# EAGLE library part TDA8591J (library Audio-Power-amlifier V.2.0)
The TDA8591J is a quad BTL audio power amplifier comprising four independent amplifiers in Bridge Tied Load (BTL) configuration. Each amplifier has a gain of 26 dB and supplies an output power of 75 W (EIAJ) into a 2 W load. The TDA8591J has low quiescent current and is primarily developed for car audio applications.
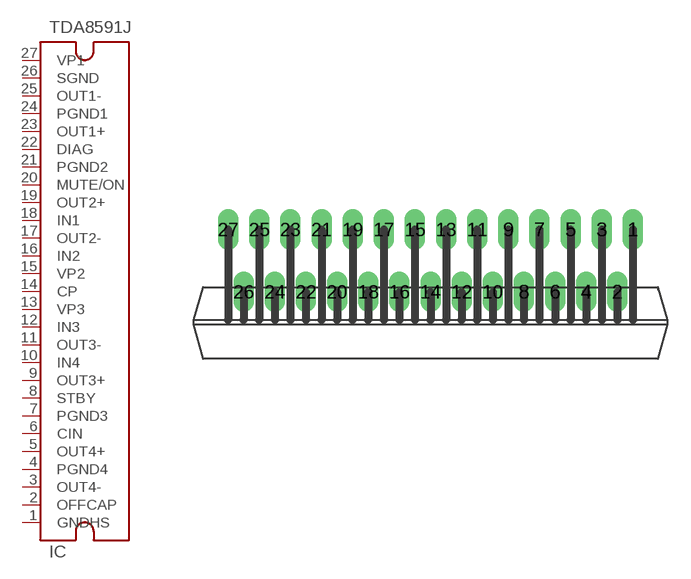
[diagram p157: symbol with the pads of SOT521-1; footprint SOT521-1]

Designator prefix IC

## TDA8591J  [SOT521-1]
1  GNDHS  pwr
2  OFFCAP
3  OUT4-  out
4  PGND4  pwr
5  OUT4+  out
6  CIN  in
7  PGND3  pwr
8  STBY  in
9  OUT3+  out
10  IN4  in
11  OUT3-  out
12  IN3  in
13  VP3  pwr
14  CP
15  VP2  pwr
16  IN2  in
17  OUT2-  out
18  IN1  in
19  OUT2+  out
20  MUTE/ON  in
21  PGND2  pwr
22  DIAG  out
23  OUT1+  out
24  PGND1  pwr
25  OUT1-  out
26  SGND  pwr
27  VP1  pwr

## Footprint SOT521-1 (pad centres in mm)
drill 0.8 long: 1 13,4; 2 12,0; 3 11,4; 4 10,0; 5 9,4; 6 8,0; 7 7,4; 8 6,0; 9 5,4; 10 4,0; 11 3,4; 12 2,0; 13 1,4; 14 0,0; 15 -1,4; 16 -2,0; 17 -3,4; 18 -4,0; 19 -5,4; 20 -6,0; 21 -7,4; 22 -8,0; 23 -9,4; 24 -10,0; 25 -11,4; 26 -12,0; 27 -13,4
